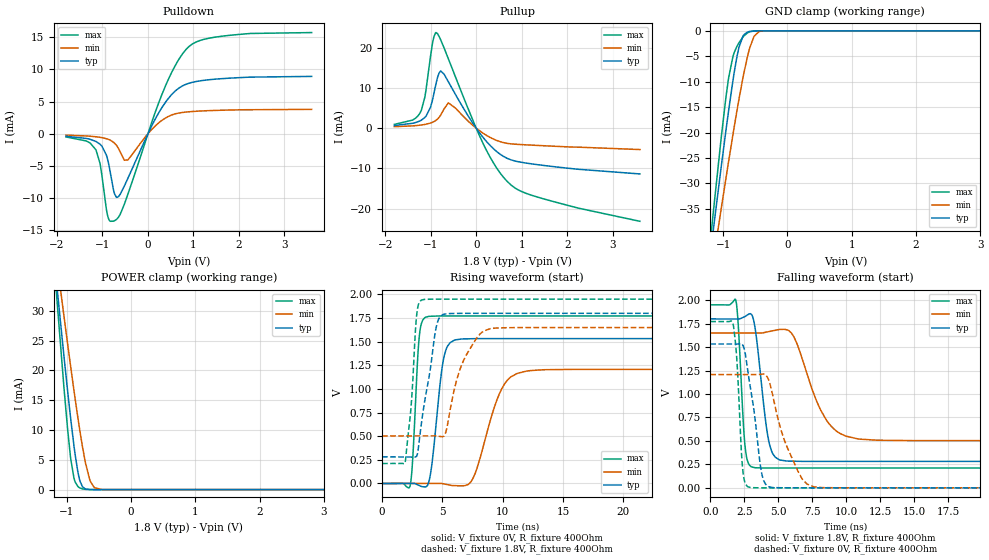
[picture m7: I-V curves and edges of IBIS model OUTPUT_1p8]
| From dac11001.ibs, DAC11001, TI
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|   OUTPUT_1p8 Model
[Model]   OUTPUT_1p8
Model_type   3-state
Polarity   Non-Inverting
Vmeas = 0.9
Vref = 0
Cref = 2pF
Rref = 100000
|   typ   min   max
C_comp   1.697pF   1.659pF   1.712pF
[Voltage Range]   1.8   1.65   1.95
[Temperature Range]   25   125   -40
[Pullup Reference]   1.8   1.65   1.95
[Pulldown Reference]   0   0   0
[Power Clamp Reference]   1.8   1.65   1.95
[GND Clamp Reference]   0   0   0
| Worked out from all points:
|   slope of the pulldown table from 0 to 0.27 V, typ, clamps not added: 73.9 ohm
|   slope of the pullup table from 0 to 0.27 V, typ, clamps not added: 70 ohm
|   GND clamp passes 1 mA (typ) near -0.69 V on its own axis
|   POWER clamp passes 1 mA (typ) near -0.78 V on its own axis
|   falling waveform, V_fixture 1.8V, R_fixture 400Ohm: 20-80 % time 714ps typ, 1.84ns min, 379ps max; typ from 1.8 V to 0.282 V
|   rising waveform, V_fixture 0V, R_fixture 400Ohm: 20-80 % time 754ps typ, 1.73ns min, 415ps max; typ from 0 V to 1.53 V
|   rising waveform, V_fixture 1.8V, R_fixture 400Ohm: 20-80 % time 1.08ns typ, 1.69ns min, 559ps max; typ from 0.282 V to 1.8 V
|   falling waveform, V_fixture 0V, R_fixture 400Ohm: 20-80 % time 842ps typ, 1.63ns min, 374ps max; typ from 1.53 V to 0 V
[Pulldown]
|   Voltage   I(typ)   I(min)   I(max)
-1.8V     -397.8uA   -219.7uA   -505.5uA
-1.147V   -1.191mA   -467.7uA   -2.475mA
-1.049V   -1.66mA    -561uA     -4.801mA
-892.8mV  -3.837mA   -820.4uA   -12.56mA
-757.8mV  -8.741mA   -1.321mA   -13.6mA
-644.4mV  -9.759mA   -2.348mA   -12.95mA
-444.6mV  -6.984mA   -4.081mA   -9.466mA
295.2mV   3.945mA    2.018mA    5.9mA
613.8mV   6.733mA    3.123mA    10.79mA
878.4mV   7.804mA    3.402mA    13.41mA
1.672V    8.594mA    3.668mA    15.21mA
3.6V      8.922mA    3.795mA    15.74mA
[GND Clamp]
|   Voltage   I(typ)   I(min)   I(max)
-1.8V     -107.4mA   -100.3mA   -119.2mA
-1.184V   -42.35mA   -47.74mA   -39.58mA
-1.141V   -37.92mA   -44.13mA   -34.24mA
-1.028V   -26.5mA    -34.77mA   -20.73mA
-914.4mV  -15.62mA   -25.62mA   -9.215mA
-849.6mV  -9.925mA   -20.55mA   -5.136mA
-757.8mV  -3.452mA   -13.71mA   -2.435mA
-693mV    -1.062mA   -9.279mA   -1.241mA
-622.8mV  -249.2uA   -5.119mA   -416.6uA
-520.2mV  -24.07uA   -1.093mA   -39.55uA
-396mV    -725.5nA   -43.8uA    -816.3nA
3.6V      0A         0A         0A
[Pullup]
|   Voltage   I(typ)   I(min)   I(max)
-1.8V     662.5uA    367.6uA    936uA
-1.4V     1.209mA    574.5uA    2.014mA
-1.211V   1.961mA    781.7uA    4.317mA
-1.125V   2.709mA    934.4uA    8.006mA
-1.006V   5.178mA    1.27mA     17.75mA
-930.6mV  8.588mA    1.63mA     22.72mA
-882mV    11.15mA    1.975mA    23.79mA
-779.4mV  14.21mA    3.268mA    21.94mA
-612mV    11.55mA    6.293mA    17.26mA
192.6mV   -2.869mA   -1.556mA   -4.771mA
765mV     -7.885mA   -3.9mA     -14.12mA
3.6V      -11.39mA   -5.318mA   -23.17mA
[POWER Clamp]
|   Voltage   I(typ)   I(min)   I(max)
-1.8V     107.6mA    94.84mA    127.7mA
-1.163V   35.3mA     39.21mA    33.51mA
-1.141V   32.94mA    37.38mA    30.48mA
-1.044V   22.55mA    29.25mA    17.33mA
-936mV    11.74mA    20.48mA    5.086mA
-876.6mV  6.517mA    15.85mA    1.544mA
-795.6mV  1.529mA    9.922mA    283.3uA
-709.2mV  110.7uA    4.53mA     42.81uA
-633.6mV  9.582uA    1.399mA    6.203uA
-568.8mV  1.321uA    305.9uA    909.6nA
-444.6mV  20.52nA    9.214uA    1.629nA
3.6V      0A         0A         0A
[Ramp]
R_load = 400
|   typ   min   max
dV/dt_r   0.919615/7.51623e-10   0.724312/1.72269e-09   1.06334/4.14791e-10
dV/dt_f   0.910813/7.13484e-10   0.688106/1.8381e-09   1.04327/3.79076e-10
[Falling Waveform]
V_fixture = 1.8V
V_fixture_min = 1.65V
V_fixture_max = 1.95V
R_fixture = 400Ohm
C_fixture = 0F
|   Time   V(typ)   V(min)   V(max)
0s        1.8V       1.65V      1.95V
1.877ns   1.799V     1.65V      2V
2.664ns   1.836V     1.649V     333.4mV
3.227ns   1.763V     1.649V     216.7mV
3.987ns   813.2mV    1.655V     211.4mV
4.791ns   325.6mV    1.679V     211.4mV
6.158ns   284.1mV    1.608V     211.4mV
9.3ns     282.2mV    603.5mV    211.4mV
14.92ns   282.2mV    503.4mV    211.4mV
3.5us     282mV      503.2mV    211.2mV
[Rising Waveform]
V_fixture = 0V
V_fixture_min = 0V
V_fixture_max = 0V
R_fixture = 400Ohm
C_fixture = 0F
|   Time   V(typ)   V(min)   V(max)
0s        944.1pV    -14.23nV   841.1pV
2.304ns   812.8uV    345.2uV    -33.58mV
3.171ns   -26.22mV   475.1uV    1.639V
3.983ns   77.1mV     596.8uV    1.768V
4.787ns   1.026V     717.1uV    1.772V
5.415ns   1.45V      -11.77mV   1.772V
7.413ns   1.531V     26.81mV    1.772V
10.55ns   1.533V     1.114V     1.772V
15.87ns   1.533V     1.207V     1.772V
3.5us     1.533V     1.207V     1.772V
[Rising Waveform]
V_fixture = 1.8V
V_fixture_min = 1.65V
V_fixture_max = 1.95V
R_fixture = 400Ohm
C_fixture = 0F
|   Time   V(typ)   V(min)   V(max)
0s        282mV      503.2mV    211.2mV
1.916ns   280mV      503.4mV    225.6mV
2.423ns   279.4mV    503.5mV    842.1mV
2.868ns   288.6mV    503.5mV    1.779V
4.282ns   1.489V     503.7mV    1.95V
5.212ns   1.792V     517.9mV    1.95V
6.429ns   1.799V     1.195V     1.95V
7.961ns   1.8V       1.558V     1.95V
11.64ns   1.8V       1.65V      1.95V
3.5us     1.8V       1.65V      1.95V
[Falling Waveform]
|Gnd
V_fixture = 0V
V_fixture_min = 0V
V_fixture_max = 0V
R_fixture = 400Ohm
C_fixture = 0F
|   Time   V(typ)   V(min)   V(max)
0s        1.533V     1.207V     1.772V
1.687ns   1.532V     1.207V     1.737V
1.95ns    1.532V     1.207V     1.375V
2.42ns    1.513V     1.207V     154mV
3.624ns   309.1mV    1.209V     156.2uV
4.291ns   12.68mV    1.152V     156.1uV
5.403ns   435uV      528.9mV    156.1uV
6.799ns   191.7uV    88.2mV     156uV
9.718ns   191.6uV    240.8uV    155.9uV
3.5us     -98.41nV   -30.92nV   -160.3nV
